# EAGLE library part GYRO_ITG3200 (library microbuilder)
ITG3200 3-Axis Digital Gyroscope VDD: 2.1-3.6V VLOGIC: 1.71V-VDD I2C Speed: 400kHz
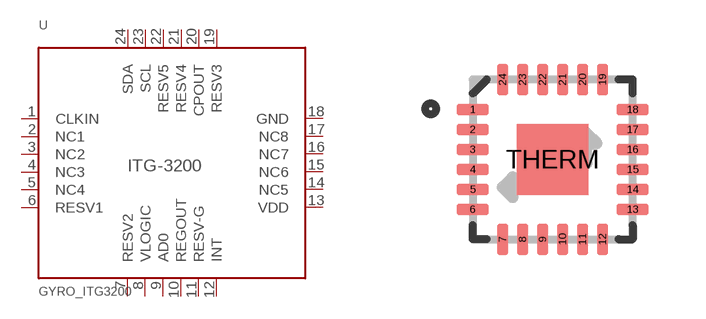
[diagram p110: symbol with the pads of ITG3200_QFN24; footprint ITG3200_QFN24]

Designator prefix U

## GYRO_ITG3200  [ITG3200_QFN24]
1  CLKIN
2  NC1
3  NC2
4  NC3
5  NC4
6  RESV1
7  RESV2
8  VLOGIC
9  AD0
10  REGOUT
11  RESV-G
12  INT
13  VDD
14  NC5
15  NC6
16  NC7
17  NC8
18  GND
19  RESV3
20  CPOUT
21  RESV4
22  RESV5
23  SCL
24  SDA

## Footprint ITG3200_QFN24 (pad centres in mm)
smd 0.8 x 0.28: 1 -2,1.25; 2 -2,0.75; 3 -2,0.25; 4 -2,-0.25; 5 -2,-0.75; 6 -2,-1.25; 13 2,-1.25; 14 2,-0.75; 15 2,-0.25; 16 2,0.25; 17 2,0.75; 18 2,1.25
smd 0.28 x 0.8: 7 -1.25,-2; 8 -0.75,-2; 9 -0.25,-2; 10 0.25,-2; 11 0.75,-2; 12 1.25,-2; 19 1.25,2; 20 0.75,2; 21 0.25,2; 22 -0.25,2; 23 -0.75,2; 24 -1.25,2
smd 1.778 x 1.778: THERM 0,0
